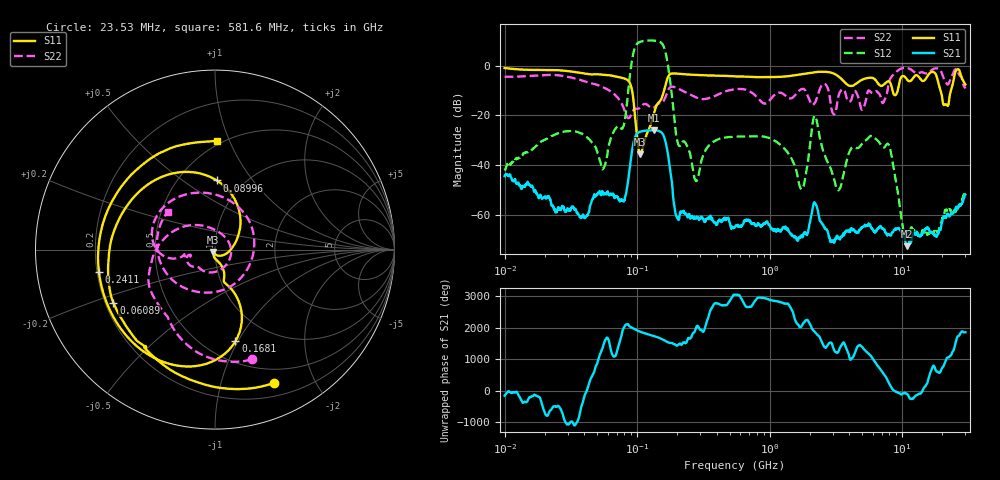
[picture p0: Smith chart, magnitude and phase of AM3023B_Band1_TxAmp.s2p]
# Hz S DB R 50.0
!freq dBS11 angS11 dBS21 angS21 dBS12 angS12 dBS22 angS22
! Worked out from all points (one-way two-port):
!   1601 points, 10 MHz to 30 GHz, reference 50 ohm
!   highest |S21| = -26.00 dB at 133.6 MHz (marker M1); lowest = -72.7 dB at 10.92 GHz (marker M2)
!   lowest |S11| = -35.7 dB at 105.6 MHz (marker M3), VSWR 1.03, Z = 49 - j1.24 ohm
!   |S11| at or under -10 dB: 91.52 MHz to 159.9 MHz (68.37 MHz wide, 54.4 % of centre); 8.44 GHz to 9.263 GHz (822.7 MHz wide, 9.3 % of centre); 19.49 GHz to 23.35 GHz (3.862 GHz wide, 18 % of centre)
!   |S22| runs from -21.2 to -0.9 dB; largest |S21 - S12| = 3.2
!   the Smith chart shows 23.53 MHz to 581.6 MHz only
!   S11 on the Smith chart (normalised r, x): 23.53 MHz: 0.34, -1.48; 60.89 MHz: 0.23, -0.23; 89.96 MHz: 0.75, +0.68; 168.1 MHz: 0.69, -0.98; 241.1 MHz: 0.21, -0.09; 581.6 MHz: 0.47, +0.90
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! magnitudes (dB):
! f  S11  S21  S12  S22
! 10 MHz  -1.0  -44.5  -42.2  -4.5
! 23.53 MHz  -1.8  -57.8  -28.0  -3.8
! 38.04 MHz  -3.0  -60.7  -27.3  -6.0
! 60.89 MHz  -3.9  -51.7  -32.5  -9.9
! 78.98 MHz  -5.1  -54.8  -24.3  -17.0
! 89.96 MHz  -8.3  -36.8  -0.4  -19.9
! 105.6 MHz  -35.7  -26.7  9.6  -16.8
! 133.6 MHz  -19.5  -26.0  10.0  -17.0
! 144.7 MHz  -14.9  -26.3  9.7  -15.3
! 168.1 MHz  -5.6  -33.6  2.3  -11.0
! 201.3 MHz  -3.3  -61.1  -30.6  -9.1
! 241.1 MHz  -3.6  -61.1  -32.9  -11.2
! 280.1 MHz  -3.8  -61.3  -46.5  -12.9
! 547.7 MHz  -4.4  -65.1  -28.6  -9.5
! 581.6 MHz  -4.4  -65.0  -28.6  -9.4
! 1.74 GHz  -3.5  -68.5  -49.8  -9.5
! 2.084 GHz  -2.9  -59.4  -25.4  -15.7
! 3.285 GHz  -4.3  -69.3  -50.2  -12.9
! 4.177 GHz  -8.2  -65.6  -33.0  -13.1
! 7.926 GHz  -6.4  -67.9  -31.9  -7.0
! 10.92 GHz  -5.7  -72.7  -67.9  -1.0
! 30 GHz  -7.6  -51.9  -50.4  -9.3
